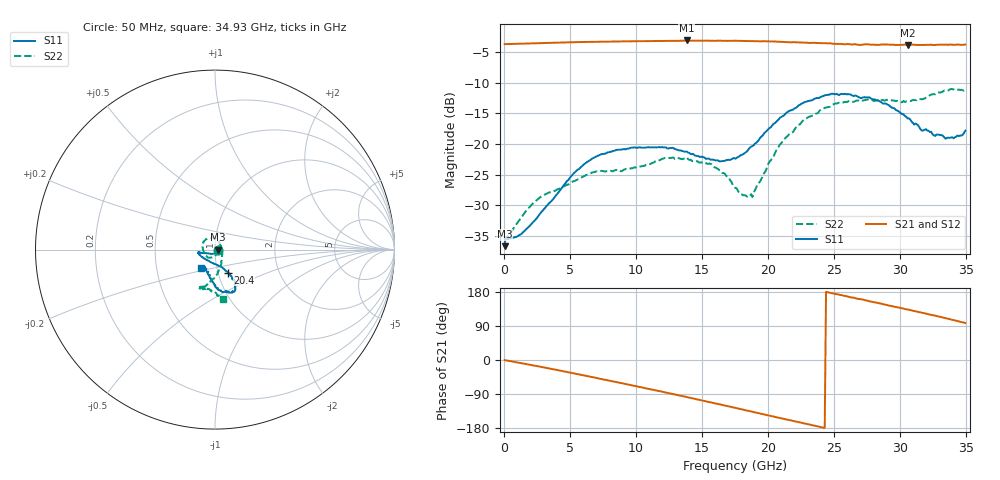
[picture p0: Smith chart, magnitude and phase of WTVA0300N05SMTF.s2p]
! 50 ohm 2-Port S-parameters measured by Modelithics Inc support@modelithics.com  Tampa, FL USA 813-866-6335 (February 2024)
! Smiths Interconnect,  3dB P/N: WTVA0300N05SMTF, Temperature: 0 C
! Board: 10 mil Rogers 4350B, Mounting Pad Dimensions: Length: 15 mils, Width: 25 mils, Gap: 40 mils.
# Hz S RI R 50
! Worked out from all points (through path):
!   352 points, 50 MHz to 34.93 GHz, reference 50 ohm
!   highest |S21| = -3.04 dB at 13.83 GHz (marker M1); lowest = -3.8 dB at 30.55 GHz (marker M2)
!   group delay of S21, straight-line fit = 21.1 ps
!   lowest |S11| = -36.7 dB at 50 MHz (marker M3), VSWR 1.03, Z = 51.5 - j0.0524 ohm
!   |S11| at or under -10 dB: start of sweep to end of sweep
!   |S22| runs from -35.6 to -11.0 dB; largest |S21 - S12| = 0.0043
!   S11 on the Smith chart (normalised r, x): 50 MHz: 1.03, -0.00; 20.4 GHz: 1.11, -0.29; 34.93 GHz: 0.84, -0.18
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5e7  0.0145 -0.000509  0.6575 -0.00299  0.6573 -0.00334  0.0175 -0.000489
1e8  0.0165 -0.00189  0.6575 -0.00661  0.6572 -0.00661  0.0164 -0.00282
1.2945e9  0.00555 -0.0174  0.6568 -0.093  0.6566 -0.093  0.00888 -0.0231
2.787e9  -0.0132 -0.024  0.6371 -0.2068  0.6366 -0.2069  0.00102 -0.0369
5.8715e9  -0.0623 -0.0196  0.5282 -0.4339  0.5278 -0.4338  -0.0275 -0.0456
8.558e9  -0.0883 -0.0153  0.36 -0.5899  0.3593 -0.5899  -0.0538 -0.0295
1.1742e10  -0.0923 -0.0201  0.0963 -0.6902  0.0954 -0.6901  -0.0701 0.0215
1.38315e10  -0.0779 -0.038  -0.0951 -0.6979  -0.0953 -0.6976  -0.0494 0.0598
1.5722e10  -0.0482 -0.0567  -0.2666 -0.6481  -0.2671 -0.6475  -0.00554 0.068
1.70155e10  -0.0232 -0.0705  -0.3743 -0.5902  -0.3747 -0.5897  0.0192 0.05
1.7513e10  -0.0113 -0.0749  -0.4153 -0.5643  -0.4156 -0.5636  0.0247 0.0359
1.88065e10  0.0244 -0.0931  -0.5058 -0.478  -0.5057 -0.4777  0.0361 -0.00686
1.92045e10  0.0378 -0.0982  -0.5297 -0.4497  -0.5298 -0.4491  0.0413 -0.023
2.03985e10  0.0708 -0.1277  -0.5931 -0.3539  -0.5932 -0.3533  0.0346 -0.07
2.11945e10  0.0891 -0.1468  -0.6224 -0.2844  -0.6222 -0.2838  0.0268 -0.1058
2.33835e10  0.1119 -0.2002  -0.6679 -0.0906  -0.6676 -0.0902  -0.0186 -0.1696
2.607e10  0.0889 -0.2402  -0.6412 0.1485  -0.6408 0.1487  -0.0761 -0.2108
2.91545e10  0.000463 -0.2068  -0.5231 0.3866  -0.5223 0.3871  -0.065 -0.2205
3.05475e10  -0.0238 -0.1601  -0.4426 0.47  -0.4413 0.4707  -0.0343 -0.2194
3.1642e10  -0.0373 -0.1229  -0.3687 0.532  -0.3686 0.5316  -0.0105 -0.2319
3.3433e10  -0.0569 -0.0946  -0.2222 0.6109  -0.2219 0.6105  0.0364 -0.2717
3.49255e10  -0.077 -0.1032  -0.0864 0.6459  -0.0835 0.6459  0.0436 -0.2728
